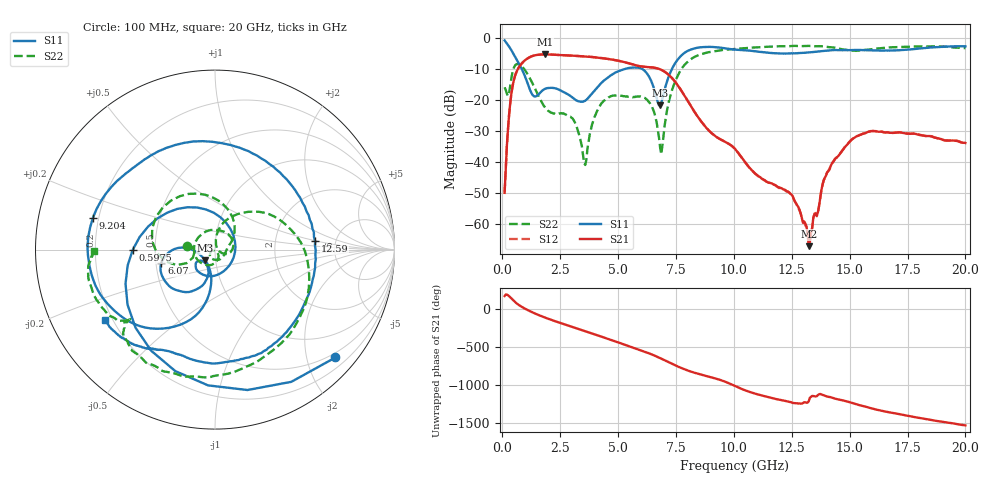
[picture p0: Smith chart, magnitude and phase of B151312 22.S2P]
!  2-Port S-parameters saved by WinCal
! VAR MeasName=S-Parameters (CALIBRATED_DATA) read from VNA (N5244A)
! VAR MeasDate=12/8/2015 5:45:07 PM
! VAR NAME=B151312 22
! VAR FILENAME=B151312 22.S2P
! VAR DATE=12/8/2015 5:45:07 PM
! VAR PHYS_PORTS=1,2
# Hz S DB R 50
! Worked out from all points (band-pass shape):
!   401 points, 100 MHz to 20 GHz, reference 50 ohm
!   highest |S21| = -5.41 dB at 1.841 GHz (marker M1); lowest = -67.3 dB at 13.23 GHz (marker M2)
!   |S21| within 3 dB of the highest: 830.9 MHz to 5.53 GHz (4.699 GHz wide, 148 % of centre)
!   lowest |S11| = -21.8 dB at 6.816 GHz (marker M3), VSWR 1.18, Z = 44.5 - j5.27 ohm
!   |S11| at or under -10 dB: 832.2 MHz to 5.342 GHz (4.509 GHz wide, 146 % of centre); 6.015 GHz to 7.334 GHz (1.319 GHz wide, 19.8 % of centre)
!   |S22| runs from -41.1 to -2.6 dB; largest |S21 - S12| = 0.0016
!   S11 on the Smith chart (normalised r, x): 100 MHz: 0.40, -2.56; 597.5 MHz: 0.37, -0.00; 6.07 GHz: 0.54, -0.09; 9.204 GHz: 0.18, +0.13; 12.59 GHz: 3.48, +0.47; 20 GHz: 0.17, -0.28
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1e8  -0.91 -41.9  -50.08 165.1  -49.91 165.2  -16.03 172.6
3.4875e8  -3.53 -122.3  -20.75 147.1  -20.74 147.0  -15.16 -154.5
5.975e8  -6.77 -179.8  -11.34 74.1  -11.34 74.1  -8.64 161.1
1.14475e9  -15.79 67.8  -6.46 -25.9  -6.46 -25.9  -12.47 73.2
1.84125e9  -16.53 -96.8  -5.41 -116.6  -5.41 -116.6  -22.45 11.7
2.53775e9  -17.10 -140.6  -5.63 169.0  -5.63 169.0  -24.36 -60.1
3.43325e9  -20.68 -128.4  -5.99 79.2  -5.98 79.2  -34.91 -158.1
3.63225e9  -20.05 -116.4  -6.08 59.2  -6.08 59.2  -39.32 -70.7
4.1795e9  -15.41 -105.7  -6.49 3.6  -6.48 3.6  -22.39 -91.8
4.92575e9  -11.12 -121.7  -7.32 -73.9  -7.32 -74.0  -18.68 177.8
6.07e9  -10.24 -166.1  -9.35 165.3  -9.36 165.1  -19.17 25.2
6.7665e9  -21.79 -149.4  -10.08 78.9  -10.09 78.9  -32.19 -21.1
6.81625e9  -21.85 -133.2  -10.22 72.0  -10.23 71.9  -35.45 -4.0
7.71175e9  -5.92 -120.6  -16.89 -55.0  -16.83 -55.2  -10.41 44.6
9.20425e9  -3.06 165.3  -31.78 165.2  -31.84 165.0  -4.33 -40.4
1.005e10  -3.87 132.1  -35.87 66.1  -35.99 65.9  -3.64 -65.5
1.258725e10  -5.03 4.8  -52.09 -156.7  -52.00 -155.7  -2.66 -113.0
1.3234e10  -4.75 -25.6  -67.29 -133.1  -66.43 -127.2  -2.66 -122.1
1.338325e10  -4.68 -32.0  -61.35 -63.4  -61.43 -64.6  -2.74 -124.2
1.437825e10  -4.02 -67.5  -39.06 -99.4  -39.02 -98.7  -3.26 -138.1
1.67165e10  -4.17 -112.3  -30.70 81.8  -30.56 82.1  -3.16 -148.0
2e10  -2.80 -147.4  -34.00 -90.0  -34.04 -91.1  -3.40 -179.2
